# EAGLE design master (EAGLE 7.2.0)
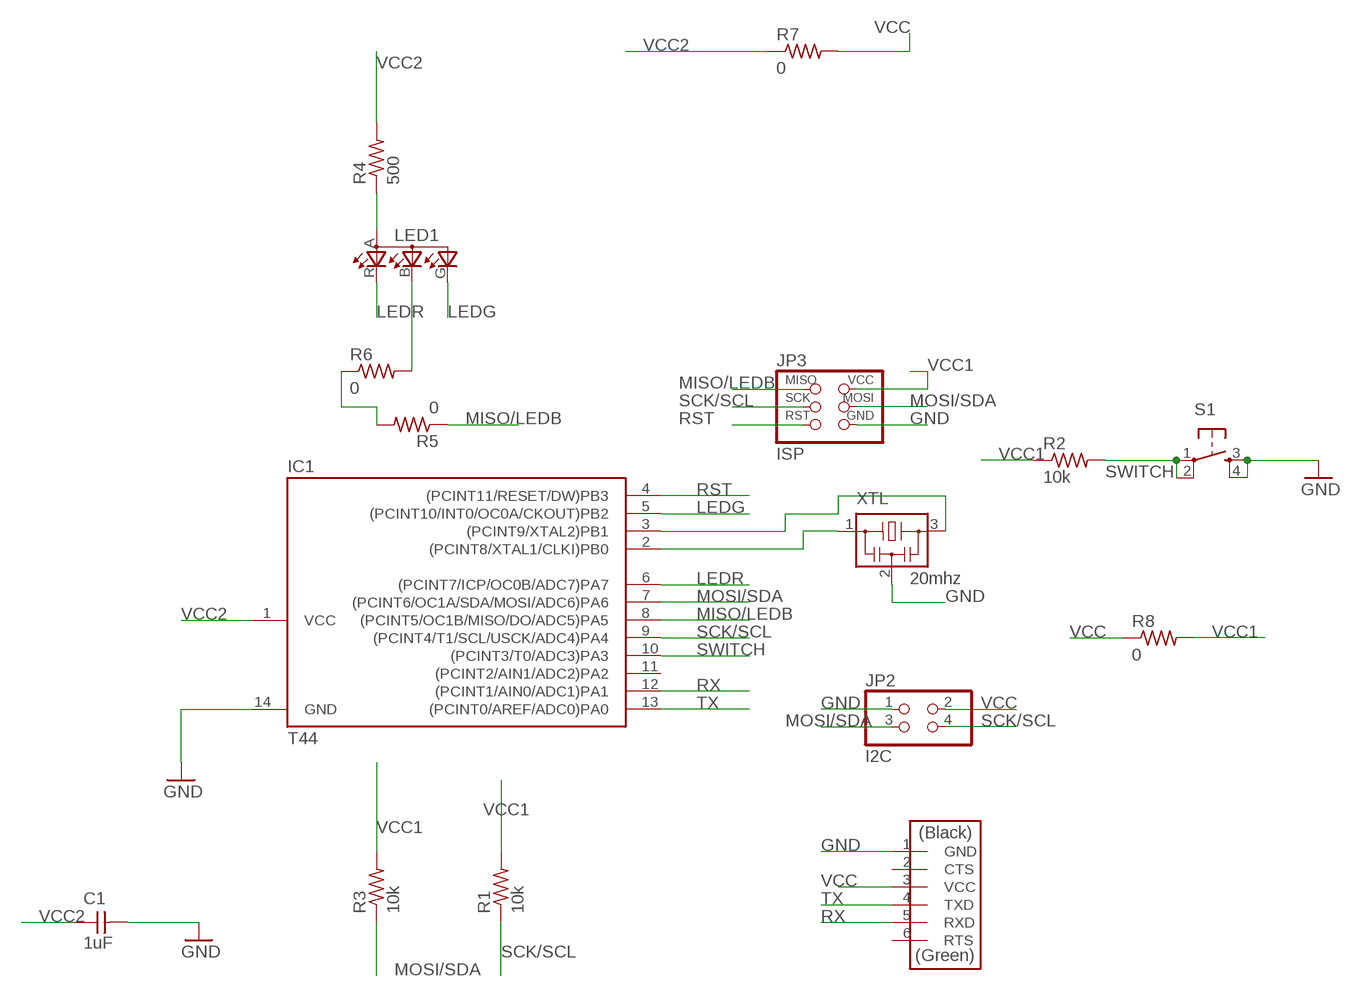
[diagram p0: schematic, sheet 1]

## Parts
C1  1uF  CAP-UNPOLARIZEDFAB  [C1206FAB]
IC1  T44  ATTINY44-SSU  [SOIC14]
JP1  FTDI  FTDI-SMD-HEADER  [1X06SMD]
JP2  I2C  PINHD-2X2-SMD  [2X02SMD]
JP3  ISP  AVRISPSMD  [2X03SMD]
LED1  LEDRGBOLD  [P-LCC-4-3]
R1  10k  RES-US1206FAB  [R1206FAB]
R2  10k  RES-US1206FAB  [R1206FAB]
R3  10k  RES-US1206FAB  [R1206FAB]
R4  500  RES-US1206FAB  [R1206FAB]
R5  0  RES-US1206FAB  [R1206FAB]
R6  0  RES-US1206FAB  [R1206FAB]
R7  0  RES-US1206FAB  [R1206FAB]
R8  0  RES-US1206FAB  [R1206FAB]
S1  6MM_SWITCH6MM_SWITCH  [6MM_SWITCH]
XTL  20mhz  RESONATOR  [EFOBM]

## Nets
GND: C1.2 IC1.14(GND) JP1.1(GND) JP2.1 JP3.6(GND) S1.3(S) S1.4(S1) XTL.2
LEDG: IC1.5((PCINT10/INT0/OC0A/CKOUT)PB2) LED1.G(CGREEN)
LEDR: IC1.6((PCINT7/ICP/OC0B/ADC7)PA7) LED1.R(CRED)
MISO/LEDB: IC1.8((PCINT5/OC1B/MISO/DO/ADC5)PA5) JP3.1(MISO) R5.1
MOSI/SDA: IC1.7((PCINT6/OC1A/SDA/MOSI/ADC6)PA6) JP2.3 JP3.4(MOSI) R3.1
N$1: LED1.A(A2) R4.1
N$2: IC1.2((PCINT8/XTAL1/CLKI)PB0) XTL.1
N$3: IC1.3((PCINT9/XTAL2)PB1) XTL.3
N$4: LED1.B(CBLUE) R6.2
N$5: R5.2 R6.1
RST: IC1.4((PCINT11/RESET/DW)PB3) JP3.5(RST)
RX: IC1.12((PCINT1/AIN0/ADC1)PA1) JP1.5(RXD)
SCK/SCL: IC1.9((PCINT4/T1/SCL/USCK/ADC4)PA4) JP2.4 JP3.3(SCK) R1.1
SWITCH: IC1.10((PCINT3/T0/ADC3)PA3) R2.2 S1.1(P) S1.2(P1)
TX: IC1.13((PCINT0/AREF/ADC0)PA0) JP1.4(TXD)
VCC: JP1.3(VCC) JP2.2 R7.2 R8.1
VCC1: JP3.2(VCC) R1.2 R2.1 R3.2 R8.2
VCC2: C1.1 IC1.1(VCC) R4.2 R7.1
Unconnected: IC1.11((PCINT2/AIN1/ADC2)PA2) JP1.2(CTS) JP1.6(RTS)

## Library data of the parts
C1 = 02fab:CAP-UNPOLARIZED
IC1 = 02fab:ATTINY44
JP1 = 02fab:FTDI-SMD-HEADER
JP2 = 02fab:PINHD-2X2-SMD
JP3 = 02fab:AVRISP
LED1 = 02fab:LEDRGBOLD: OSRAM Hyper Multi TOPLED® Hyper-Bright LED LATB T686 Source: http://www.osram.convergy.de/
R1-R8 = 02fab:RES-US: Resistor (US Symbol)
S1 = 02fab:6MM_SWITCH: OMRON SWITCH
XTL = 02fab:RESONATOR

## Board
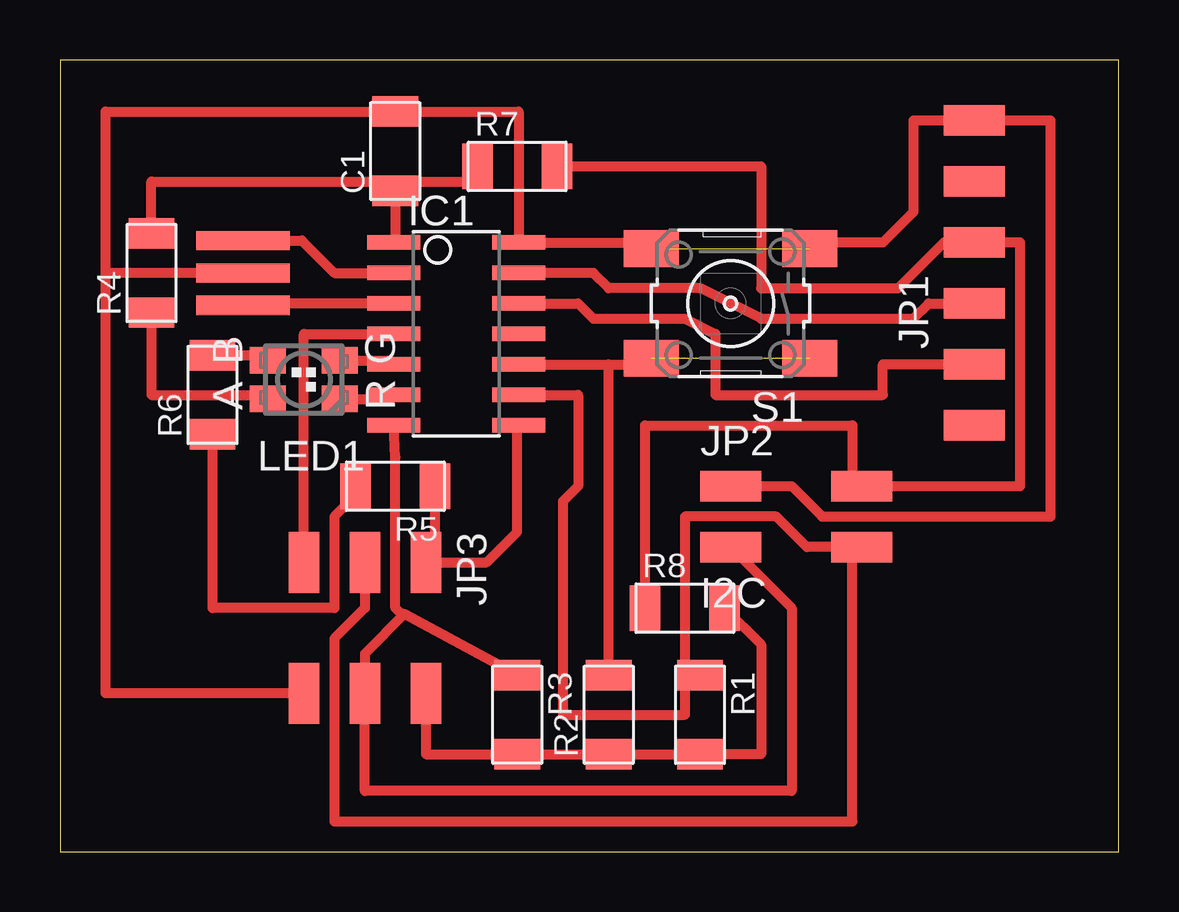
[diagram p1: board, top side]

Size 44.12 x 33.01 mm. Coordinates in mm from the lower left corner, seen from the top.
Outline: 0,0 44.12,0 44.12,33.01 0,33.01 0,0
Copper layers (1*16): Top 0.035mm / dielectric 1.5mm / Bottom 0.035mm
Design rules "default": minimum track width 10mil, minimum drill 24mil, track to track 8mil, track to pad 8mil, pad to pad 8mil, via to via 8mil, smd to smd 8mil, copper to edge 40mil, drill to drill 8mil, minimum pad ring 10mil, minimum via ring 8mil, stop-mask expansion 4mil, vias tented up to drill 0mil, thermal gap 10mil

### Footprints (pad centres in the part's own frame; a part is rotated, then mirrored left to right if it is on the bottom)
C1206FAB = smd 1.27 x 1.905: 1 -1.651,0; 2 1.651,0
SOIC14 = smd 0.61 x 2.21: 1 -3.81,-2.603; 2 -2.54,-2.603; 3 -1.27,-2.603; 4 0,-2.603; 5 1.27,-2.603; 6 2.54,-2.603; 7 3.81,-2.603; 8 3.81,2.603; 9 2.54,2.603; 10 1.27,2.603; 11 0,2.603; 12 -1.27,2.603; 13 -2.54,2.603; 14 -3.81,2.603
1X06SMD = smd 2.54 x 1.27: 1 0,6.35; 2 0,3.81; 3 0,1.27; 4 0,-1.27; 5 0,-3.81; 6 0,-6.35
2X02SMD = smd 2.54 x 1.27: 1 -2.54,1.27; 2 2.92,1.27; 3 -2.54,-1.27; 4 2.92,-1.27
2X03SMD = smd 2.54 x 1.27: 1 -2.54,2.54; 2 2.92,2.54; 3 -2.54,0; 4 2.92,0; 5 -2.54,-2.54; 6 2.92,-2.54
P-LCC-4-3 = smd 1.1 x 1.5: A -0.8,1.5; B 0.8,1.5; G 0.8,-1.5; R -0.8,-1.5
R1206FAB = smd 1.27 x 1.905: 1 -1.651,0; 2 1.651,0
6MM_SWITCH = smd 2.286 x 1.524: 1 -3.302,2.286; 2 3.302,2.286; 3 -3.302,-2.286; 4 3.302,-2.286
EFOBM = smd 0.8 x 3.9: 1 -1.35,0; 2 0,0; 3 1.35,0

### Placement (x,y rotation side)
C1  13.97,29.21 90 top
IC1  16.51,21.59 270 top
JP1  38.1,24.13 0 top
JP2  30.48,13.97 0 top
JP3  12.7,9.53 270 top
LED1  10.16,19.68 90 top
R1  26.67,5.71 270 top
R2  22.86,5.71 90 top
R3  19.05,5.71 270 top
R4  3.81,24.13 90 top
R5  13.97,15.24 180 top
R6  6.35,19.05 90 top
R7  19.05,28.57 0 top
R8  26.04,10.16 0 top
S1  27.94,22.86 180 top
XTL  7.62,24.13 270 top

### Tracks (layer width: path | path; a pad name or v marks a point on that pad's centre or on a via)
GND  (1 unrouted)
  Top 0.406: XTL.2 1.9,24.13 | 19.05,25.46 IC1.14 | 1.9,24.13 1.9,6.61 JP3.6 | IC1.14 24.38,25.4 S1.4 25.4,25.15 | JP2.1 30.48,15.24 31.75,13.97 41.27,13.97 41.27,30.48 JP1.1 35.56,30.48 35.56,26.67 34.29,25.4 31.5,25.4 S1.3 31.75,25.15 | 1.9,24.13 1.9,30.86 C1.2 19.11,30.86 IC1.14
LEDG
  Top 0.406: LED1.G 13.74,20.48 IC1.5
LEDR
  Top 0.406: LED1.R 13.74,18.89 IC1.6
MISO/LEDB
  Top 0.406: IC1.8 19.05,17.72 19.05,13.34 17.78,12.07 JP3.1 15.62,12.45 R5.1
MOSI/SDA
  Top 0.406: R3.1 14.35,9.91 | 14.35,9.91 12.7,8.26 JP3.4 12.7,2.54 30.48,2.54 30.48,10.16 JP2.3 | 14.35,9.91 14.22,9.91 13.97,10.16 13.97,16.45 IC1.7
N$1
  Top 0.406: R4.1 3.81,19.05 8.5,19.05 LED1.A
N$2
  Top 0.406: XTL.1 10.08,25.48 11.43,24.13 IC1.2
N$3
  Top 0.406: IC1.3 7.7,22.86 XTL.3
N$4
  Top 0.406: R6.2 8.44,20.7 LED1.B
N$5
  Top 0.406: R5.2 12.32,14.86 11.43,13.97 11.43,10.16 6.35,10.16 R6.1
RST
  Top 0.406: JP3.5 10.16,21.59 IC1.4
RX
  Top 0.406: IC1.12 21.59,22.86 22.23,22.23 26.04,22.23 27.3,21.59 27.3,19.05 34.29,19.05 34.29,20.32 JP1.5
SCK/SCL
  Top 0.406: IC1.9 21.59,19.05 21.59,15.24 20.96,14.61 20.96,5.71 26.04,5.71 26.04,7.62 | JP3.3 12.7,10.16 11.43,8.89 11.43,1.27 33.02,1.27 33.02,12.7 JP2.4 | 26.04,7.62 26.04,13.97 29.84,13.97 31.11,12.7 JP2.4 | R1.1 26.67,7.62 26.04,7.62 | 33.65,12.7 JP2.4
SWITCH  (1 unrouted)
  Top 0.406: IC1.10 22.86,20.32 | 22.86,20.32 24.38,20.32 S1.2 | R2.2 22.86,20.32
TX
  Top 0.406: IC1.13 22.23,24.13 22.86,23.5 26.67,23.5 29.21,22.23 35.56,22.23 36.2,22.86 JP1.4
VCC
  Top 0.406: R8.1 24.38,17.78 33.02,17.78 33.02,15.24 JP2.2 40,15.24 40,25.4 JP1.3 36.83,25.4 34.92,23.5 29.21,23.5 29.21,28.57 R7.2
VCC1
  Top 0.406: JP3.2 15.24,4.06 R3.2 R2.1 R1.2 29.21,4.06 29.21,8.64 R8.2
VCC2
  Top 0.406: R4.2 3.81,27.94 13.97,27.94 | 13.97,27.94 C1.1 13.97,25.4 IC1.1 | 13.97,27.94 17.4,27.94 R7.1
